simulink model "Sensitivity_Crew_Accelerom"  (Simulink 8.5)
settings: Solver=ode45  StartTime=0.0  StopTime=100000  RelTol=1e-3
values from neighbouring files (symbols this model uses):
  Kpqr = lqr(sys,Q0,R0)    [des.m]
  wo = 0.0011    [start.m]    (also in start1.m; start2.m; start3.m)
undefined symbols (not defined in the file or in its folder): Af, Bf, Cf, Df

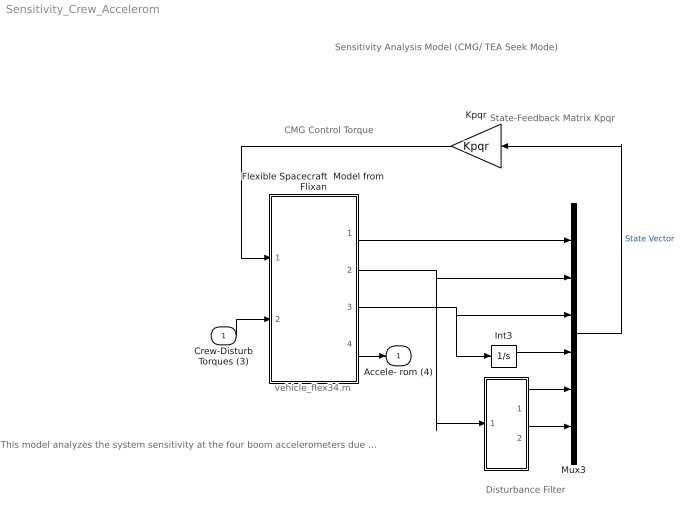
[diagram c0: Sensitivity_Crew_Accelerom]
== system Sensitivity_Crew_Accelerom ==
  note: Sensitivity Analysis Model (CMG/ TEA Seek Mode)
  note: State-Feedback Matrix Kpqr
  note: CMG Control Torque
  note: Disturbance Filter
  note: vehicle_flex34.m
  note: This model analyzes the system sensitivity at the four boom accelerometers due to disturbance torques Td (x,y,z) coming from the crew compartment. The aero disturbances are being ignored
  Crew-Disturb Torques (3) : Inport
  " " : Subsystem
  Flexible Spacecraft  Model from Flixan : Subsystem
  Int3 : Integrator
  Kpqr : Gain  Gain=Kpqr  Multiplication=Matrix(K*u)
  Mux3 : Mux  Inputs=[3, 3, 3, 3, 1, 1]
  Accele- rom (4) : Outport
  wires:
  Int3/1 -> Mux3/4
  Kpqr/1 -> Flexible Spacecraft  Model from Flixan/1(Tcmg)
  Mux3/1 -> Kpqr/1  "State Vector"
  " "/1(a1) -> Mux3/5
  " "/2(a2) -> Mux3/6
  Flexible Spacecraft  Model from Flixan/3("Hcmg ") -> Int3/1, Mux3/3
  Flexible Spacecraft  Model from Flixan/2(att-lv) -> " "/1(the), Mux3/2
  Flexible Spacecraft  Model from Flixan/1(w-lv) -> Mux3/1
  Flexible Spacecraft  Model from Flixan/4(4 accel) -> Accele- rom (4)/1
  Crew-Disturb Torques (3)/1 -> Flexible Spacecraft  Model from Flixan/2(Crew-Dist)

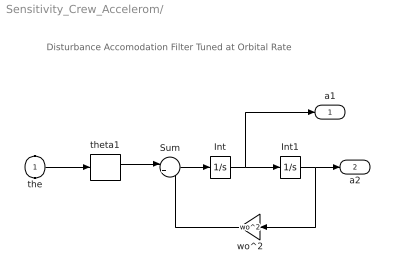
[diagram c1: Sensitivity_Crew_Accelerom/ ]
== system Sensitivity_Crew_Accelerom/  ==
  note: Disturbance Accomodation Filter Tuned at Orbital Rate
  the : Inport
  Int : Integrator
  Int1 : Integrator
  Sum : Sum  Inputs=|+-
  theta1 : Selector  InputPortWidth=3  Indices=[2]
  wo^2 : Gain  Gain=wo^2
  a1 : Outport
  a2 : Outport  Port=2
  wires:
  Int/1 -> Int1/1, a1/1
  Sum/1 -> Int/1
  Int1/1 -> wo^2/1, a2/1
  wo^2/1 -> Sum/2
  theta1/1 -> Sum/1
  the/1 -> theta1/1

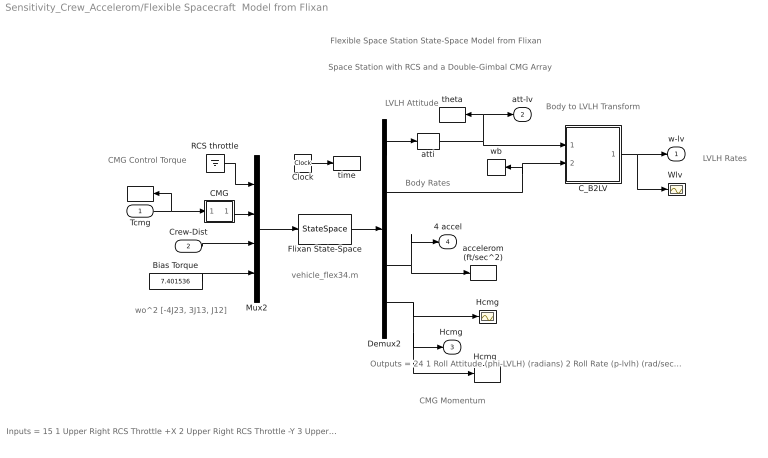
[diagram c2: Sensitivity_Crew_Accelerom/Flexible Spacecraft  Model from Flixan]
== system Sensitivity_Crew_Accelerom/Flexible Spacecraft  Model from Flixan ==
  note: Flexible Space Station State-Space Model from Flixan
  note: Space Station with RCS and a Double-Gimbal CMG Array
  note: wo^2 [-4J23, 3J13, J12]
  note: Inputs = 15 1 Upper Right RCS Throttle +X 2 Upper Right RCS Throttle -Y 3 Upper Left RCS Throttle +X 4 Upper Left RCS Throttle +Y 5 Lower Right RCS Throttle +X 6 Lower Right RCS Throttle -Y 7 Lower Left RCS Throttle +X 8 Lower Left RCS Throttle +Y 9 Double Gimbal CMG Torque in the X-axis (ft-lb) 10 Double Gimbal CMG Torque in the Y-axis (ft-lb) 11 Double Gimbal CMG Torque in the Z-axis (ft-lb) 12 External Torque Input 1 (ft-lb), direct: 13 External Torque Input 2 (ft-lb), direct: 14 External Torque Input 3 (ft-lb), direct: 15 Ext Torque Direct.=(0.197, -0.5964, -0.7782)
  note: CMG Momentum
  note: LVLH Attitude
  note: LVLH Rates
  note: Body to LVLH Transform
  note: Body Rates
  note: CMG Control Torque
  note: vehicle_flex34.m
  note: Outputs = 24 1 Roll Attitude (phi-LVLH) (radians) 2 Roll Rate (p-lvlh) (rad/sec) 3 Pitch Attitude (thet-LVLH) (radians) 4 Pitch Rate (q-lvlh) (rad/sec) 5 Yaw Attitude (psi-LVLH) (radians) 6 Yaw Rate (r-lvlh) (rad/sec) 7 Angle of attack, alfa, (radians) 8 Angle of sideslip, beta, (radian) 9 Change in Altitude, delta-h, (feet) 10 Forward Acceleration (V-dot) (ft/sec) 11 Cross Range Velocity (Vcr) (ft/sec) 12 Rate-Gyro # 1, Roll Rate (Body) (rad/sec) 13 Rate-Gyro # 2, Pitch Rate (Body) (rad/sec) 14 Rate-Gyro # 3, Yaw Rate (Body) (rad/sec) 15 Gyro # 4, Roll Attitude (Body) (radians) 16 Gyro # 5, Pitch Attitude (Body) (radians) 17 Gyro # 6, Yaw Attitude (Body) (radians) 18 Accelerom # 1, (along X), (ft/sec^2) Translat. Accelerat. 19 Accelerom # 2, (along Z), (ft/sec^2) Translat. Accelerat. 20 Accelerom # 3, (along X), (ft/sec^2) Translat. Accelerat. 21 Accelerom # 4, (along Z), (ft/sec^2) Translat. Accelerat. 22 Double Gimbal CMG Momentum Change in X-axis (ft-lb-sec) 23 Double Gimbal CMG Momentum Change in Y-axis (ft-lb-sec) 24 Double Gimbal CMG Momentum Change in Z-axis (ft-lb-sec)
  Tcmg : Inport  PortDimensions=3
  Crew-Dist : Inport  Port=2  PortDimensions=3
  "   " : ToWorkspace  VariableName=Tcmg  SampleTime=-1
  Bias Torque : Constant  Value=7.401536
  CMG : Subsystem
  C_B2LV : Subsystem
  Clock : Clock
  Demux2 : Demux  Outputs=[11, 3, 3, 4, 3]
  Flixan State-Space : StateSpace  A=Af  B=Bf  C=Cf  D=Df  X0=0
  Hcmg : Scope
  "Hcmg  " : ToWorkspace  VariableName=Hcmg  SampleTime=-1
  Mux2 : Mux  Inputs=[8, 3, 3, 1]
  RCS throttle : Ground
  "Wlv " : Scope
  accelerom (ft/sec^2) : ToWorkspace  VariableName=accel  SampleTime=-1
  atti : Selector  InputPortWidth=11  Indices=[1 3 5]
  theta : ToWorkspace  VariableName=theta  SampleTime=-1
  time : ToWorkspace  VariableName=time  SampleTime=-1
  wb : ToWorkspace  VariableName=wb  SampleTime=-1
  w-lv : Outport
  att-lv : Outport  Port=2
  "Hcmg " : Outport  Port=3
  4 accel : Outport  Port=4
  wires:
  Mux2/1 -> Flixan State-Space/1
  Flixan State-Space/1 -> Demux2/1
  Bias Torque/1 -> Mux2/4
  Clock/1 -> time/1
  RCS throttle/1 -> Mux2/1
  Demux2/5 -> Hcmg/1, "Hcmg "/1, "Hcmg  "/1
  Demux2/1 -> atti/1
  Demux2/4 -> accelerom (ft/sec^2)/1, 4 accel/1
  Tcmg/1 -> CMG/1(I), "   "/1
  Crew-Dist/1 -> Mux2/3
  CMG/1(O) -> Mux2/2
  atti/1 -> theta/1, att-lv/1, C_B2LV/1(atti)
  Demux2/2 -> C_B2LV/2(wb), wb/1
  C_B2LV/1(wlv) -> "Wlv "/1, w-lv/1

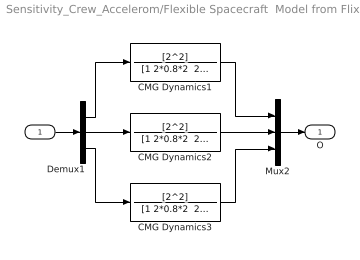
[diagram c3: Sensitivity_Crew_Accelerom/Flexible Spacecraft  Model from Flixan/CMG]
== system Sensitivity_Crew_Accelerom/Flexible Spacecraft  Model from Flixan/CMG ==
  I : Inport
  CMG Dynamics1 : TransferFcn  Numerator=[2^2]  Denominator="[1 2*0.8*2  2^2]"
  CMG Dynamics2 : TransferFcn  Numerator=[2^2]  Denominator="[1 2*0.8*2  2^2]"
  CMG Dynamics3 : TransferFcn  Numerator=[2^2]  Denominator="[1 2*0.8*2  2^2]"
  Demux1 : Demux  Outputs=3
  Mux2 : Mux  Inputs=3
  O : Outport
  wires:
  Mux2/1 -> O/1
  I/1 -> Demux1/1
  Demux1/3 -> CMG Dynamics3/1
  Demux1/1 -> CMG Dynamics1/1
  Demux1/2 -> CMG Dynamics2/1
  CMG Dynamics1/1 -> Mux2/1
  CMG Dynamics3/1 -> Mux2/3
  CMG Dynamics2/1 -> Mux2/2

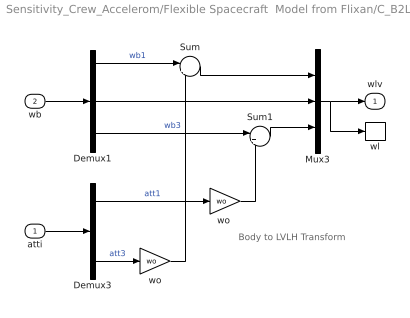
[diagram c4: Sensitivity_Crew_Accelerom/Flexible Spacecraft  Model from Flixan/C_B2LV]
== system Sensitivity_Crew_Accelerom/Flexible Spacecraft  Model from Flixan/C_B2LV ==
  note: Body to LVLH Transform
  atti : Inport  PortDimensions=3
  wb : Inport  Port=2  PortDimensions=3
  Demux1 : Demux  Outputs=3
  Demux3 : Demux  Outputs=3
  Mux3 : Mux  Inputs=3
  Sum : Sum  Inputs=|++
  Sum1 : Sum  Inputs=|+-
  wl : ToWorkspace  VariableName=wl  SampleTime=-1
  wo : Gain  Gain=wo
  "wo " : Gain  Gain=wo
  wlv : Outport
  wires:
  "wo "/1 -> Sum1/2
  Demux1/3 -> Sum1/1  "wb3"
  wo/1 -> Sum/2
  Demux1/2 -> Mux3/2
  Demux3/1 -> "wo "/1  "att1"
  Mux3/1 -> wl/1, wlv/1
  wb/1 -> Demux1/1
  atti/1 -> Demux3/1
  Sum1/1 -> Mux3/3
  Demux3/3 -> wo/1  "att3"
  Sum/1 -> Mux3/1
  Demux1/1 -> Sum/1  "wb1"
